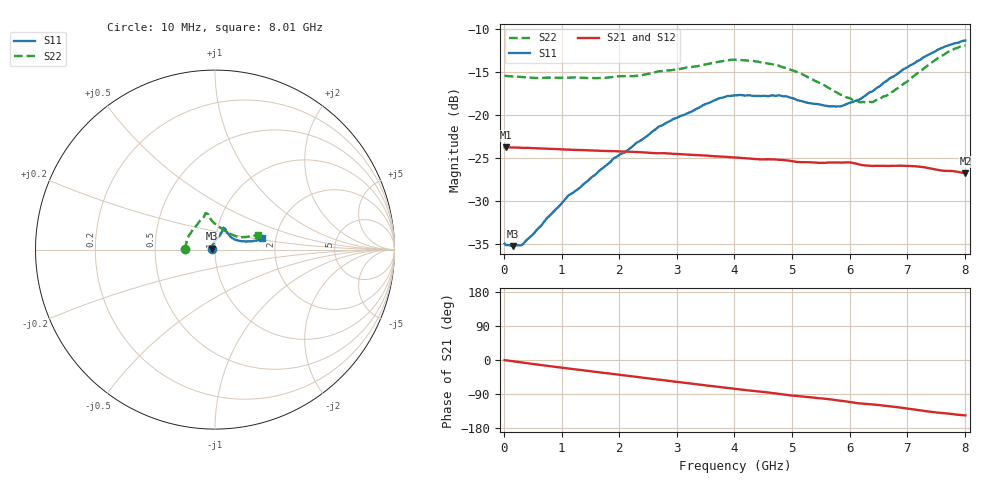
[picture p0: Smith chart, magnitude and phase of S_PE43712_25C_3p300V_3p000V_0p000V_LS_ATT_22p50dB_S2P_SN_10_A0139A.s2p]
! DEVICE ID: PE43712
! File Path: z:\PE43713\PE43713_CHAR_NOM_04292014\AMB\3p300\LS_ATT_22p50dB\PE43713_AMB_3p300V_3p000V_0p000V_LS_ATT_22p50dB_S2P_SN_10_A0139A.s2p
! Serial: 10
! Lot: A0139A
! Temp: 25C
! VDD: 3.300
! VSS: 0.000
! Control_Hi: 3.000
! Control_Lo: 0.000
! Attenuation Step: 22.50dB
! Port 1: RF1
! Port 2: RF2
! ThroughPath:1-2
! IDD: 0.0001469981
! ISS: -7.97e-008
#  Hz  S  RI  R  50
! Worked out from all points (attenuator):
!   801 points, 10 MHz to 8.01 GHz, reference 50 ohm
!   highest |S21| = -23.74 dB at 30 MHz (marker M1); lowest = -26.8 dB at 8.01 GHz (marker M2)
!   lowest |S11| = -35.2 dB at 160 MHz (marker M3), VSWR 1.04, Z = 48.4 + j0.523 ohm
!   |S11| at or under -10 dB: start of sweep to end of sweep
!   |S22| runs from -18.5 to -11.9 dB; largest |S21 - S12| = 0.00025
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1e7  -0.0179 0.00068  0.065 -0.000308  0.065 -0.000307  -0.1692 0.00117
3e7  -0.0175 0.00166  0.065 -0.000786  0.065 -0.000785  -0.1687 0.00294
1.6e8  -0.0164 0.00541  0.0647 -0.0039  0.0647 -0.0039  -0.1671 0.0117
3.3e8  -0.0149 0.0097  0.064 -0.00787  0.064 -0.00779  -0.1647 0.0215
1.11e9  -0.01 0.0324  0.0582 -0.0239  0.0583 -0.0239  -0.1501 0.0681
1.35e9  -0.00637 0.0383  0.0559 -0.0282  0.0559 -0.0282  -0.1436 0.0804
1.91e9  0.00515 0.0559  0.0491 -0.0373  0.0491 -0.0373  -0.1228 0.1132
2.34e9  0.0167 0.0681  0.0428 -0.0434  0.0427 -0.0434  -0.1035 0.1341
2.68e9  0.0272 0.0809  0.0373 -0.047  0.0373 -0.047  -0.087 0.157
3.71e9  0.0448 0.1156  0.019 -0.0542  0.019 -0.0542  -0.0559 0.1954
4.01e9  0.0473 0.1214  0.0137 -0.055  0.0136 -0.055  -0.0532 0.2027
4.31e9  0.0478 0.1202  0.00846 -0.055  0.00847 -0.0551  -0.0459 0.2012
4.75e9  0.0541 0.1181  0.000901 -0.0551  0.000983 -0.0551  -0.0353 0.1911
5.35e9  0.0685 0.0943  -0.00829 -0.0524  -0.00828 -0.0524  -0.018 0.1607
5.82e9  0.0875 0.0701  -0.0156 -0.0506  -0.0155 -0.0507  0.0155 0.1315
6.17e9  0.1095 0.056  -0.0214 -0.0469  -0.0213 -0.047  0.0497 0.1081
6.4e9  0.1277 0.0512  -0.0232 -0.045  -0.0231 -0.045  0.0752 0.0921
6.68e9  0.155 0.0465  -0.0267 -0.043  -0.0266 -0.043  0.1079 0.0772
7.15e9  0.1977 0.0457  -0.0332 -0.0379  -0.0331 -0.0378  0.1573 0.0698
7.56e9  0.2364 0.0521  -0.0362 -0.0312  -0.0362 -0.0312  0.2034 0.0754
7.81e9  0.2537 0.058  -0.0378 -0.0283  -0.0378 -0.0283  0.2275 0.0816
8.01e9  0.2637 0.0632  -0.038 -0.0255  -0.038 -0.0256  0.2391 0.083
